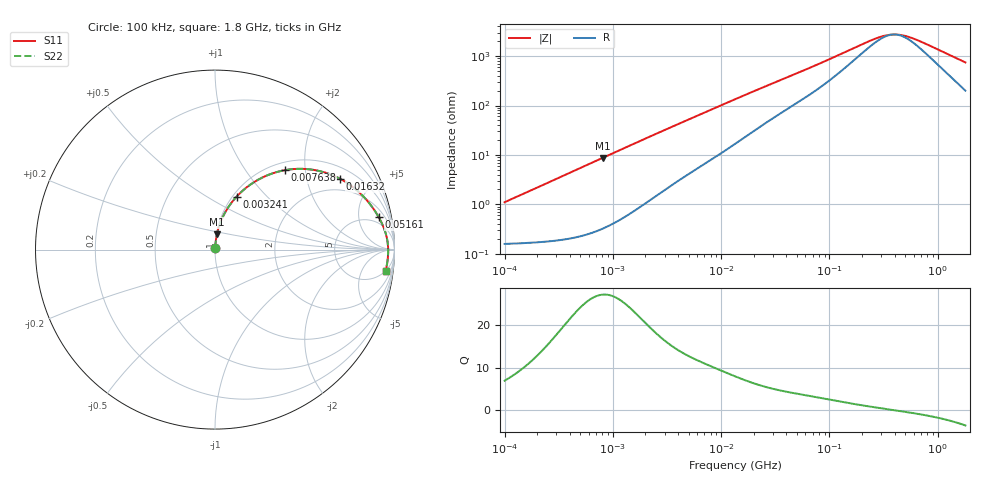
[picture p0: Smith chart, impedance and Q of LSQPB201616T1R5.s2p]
! LSQPB201616T1R5  S-PARAMETER MODEL  ( General Type )
! Model Generated by TAIYO YUDEN Corporation (http://www.ty-top.com)
! Version 2.0
! TAIYO YUDEN Control No. 100810NC14SB-FKC
! Copyright(c) 2008 TAIYO YUDEN CO.,LTD. All Rights Reserved.
! Product Description (link to TY-COMPAS)
! https://ds.yuden.co.jp/TYCOMPAS/or/detail?pn=LSQPB201616T1R5M&u=M
! Products Name : Inductors
! Characteristics :
!  Inductance : 1.5 uH , SRF(min) : 370 MHz , DC Resistance(max) : 0.195 Ohm
!  Rated Current : Saturation :1100 mA , Temp Rise : 820 mA (40 degC)
!  Case Size : 2.0 x 1.6 / 0.079 x 0.063 [mm/inch] , Thickness : 1.6 / 0.063 [mm/inch]
!  (Conditions: Temperature = 25 degC , DC Bias Current/Voltage = 0A / 0V)
! External Node Assignments :
!  1  o---GGG---o  2
! GND o---------o GND
! Frequency Range : 0.1MHz  -  1800MHz  [ 402 STEP ]
# MHz S RI R 50
! Freq[MHz].  S11 Real  S11 Imag  S21 Real  S21 Imag  S12 Real  S12 Imag  S22 Real  S22 Imag
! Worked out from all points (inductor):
!   401 points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, 100 kHz to 1.8 GHz, reference 50 ohm
!   read as one part in series: L = 1.73 uH near 105 kHz
!   highest Q = 27.1 at 802.1 kHz (marker M1), where L = 1.72 uH
!   self-resonance near 394.4 MHz
!   S11 on the Smith chart (normalised r, x): 100 kHz: 1.00, +0.02; 3.241 MHz: 1.04, +0.68; 7.638 MHz: 1.15, +1.55; 16.32 MHz: 1.45, +3.19; 51.61 MHz: 3.34, +8.94; 1.8 GHz: 5, -14
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0.1  0.00169 0.0109  0.9983 -0.0109  0.9983 -0.0109  0.00169 0.0109
0.516129  0.00537 0.0555  0.9946 -0.0555  0.9946 -0.0555  0.00537 0.0555
0.802131  0.0106 0.0855  0.9894 -0.0855  0.9894 -0.0855  0.0106 0.0855
1.592628  0.0352 0.1639  0.9648 -0.1639  0.9648 -0.1639  0.0352 0.1639
2.66389  0.0868 0.2544  0.9132 -0.2544  0.9132 -0.2544  0.0868 0.2544
3.240572  0.1201 0.2948  0.8799 -0.2948  0.8799 -0.2948  0.1201 0.2948
4.914404  0.225 0.3804  0.775 -0.3804  0.775 -0.3804  0.225 0.3804
7.637621  0.3889 0.4425  0.6111 -0.4425  0.6111 -0.4425  0.3889 0.4425
9.999495  0.5047 0.4491  0.4953 -0.4491  0.4953 -0.4491  0.5047 0.4491
13.41641  0.6261 0.4251  0.3739 -0.4251  0.3739 -0.4251  0.6261 0.4251
16.32081  0.6966 0.3947  0.3034 -0.3947  0.3034 -0.3947  0.6966 0.3947
27.2988  0.829 0.2936  0.171 -0.2936  0.171 -0.2936  0.829 0.2936
51.61028  0.912 0.181  0.088 -0.181  0.088 -0.181  0.912 0.181
69.24595  0.9327 0.1399  0.0673 -0.1399  0.0673 -0.1399  0.9327 0.1399
124.6553  0.9548 0.0765  0.0452 -0.0765  0.0452 -0.0765  0.9548 0.0765
247.5026  0.9634 0.0266  0.0366 -0.0266  0.0366 -0.0266  0.9634 0.0266
301.0823  0.9643 0.0151  0.0357 -0.0151  0.0357 -0.0151  0.9643 0.0151
357.3983  0.9647 0.00545  0.0353 -0.00545  0.0353 -0.00545  0.9647 0.00545
445.5497  0.9649 -0.00676  0.0351 0.00676  0.0351 0.00676  0.9649 -0.00676
569.2172  0.9646 -0.0208  0.0354 0.0208  0.0354 0.0208  0.9646 -0.0208
727.2099  0.9638 -0.036  0.0362 0.036  0.0362 0.036  0.9638 -0.036
1800  0.9505 -0.1185  0.0495 0.1185  0.0495 0.1185  0.9505 -0.1185
